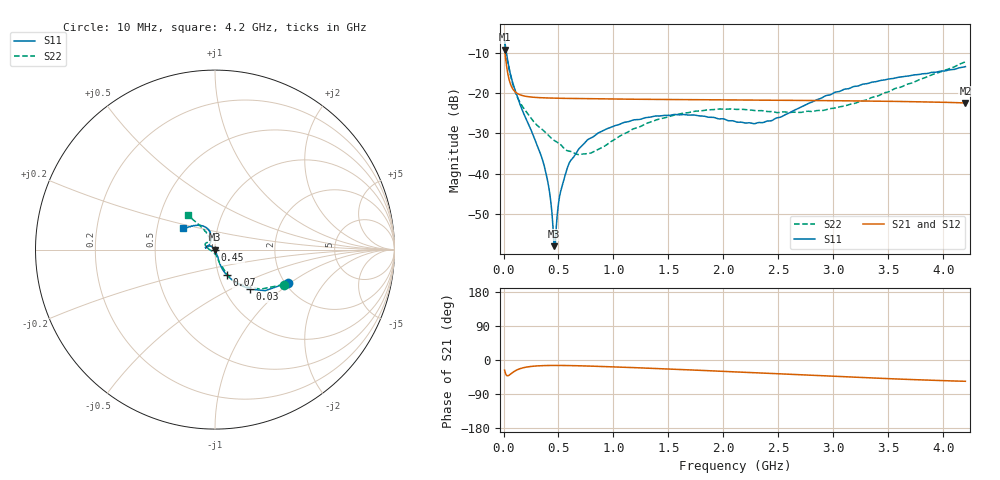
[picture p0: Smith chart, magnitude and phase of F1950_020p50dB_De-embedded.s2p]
! Integrated Device Technology
! Corporate Headquarters
! 6024 Silver Creek Valley Road
! San Jose, CA 95138  USA
! Phone:  1-408-284-8200
! Toll Free:  1-800-223-1366
! Webpage:  http://www.idt.com/
! Timing and RF Division
! 515 Groton Road, Suite 102
! Westford, MA 01886-6024
! Device:  F1950
! Description: 7-bit 0.25 dB Digital Step Attenuator
! Frequency:  150.0 -  4000.00 MHz
! Package:  4x4 mm Thin QFN Plastic Package: 24 pin
! Ports:  2 RF, 12 DC
!  Pin  1  = D0
!  Pin  2  = VDD
!  Pin  3  = Vmode
!  Pin  4  = GND
!  Pin  5  = RF1  =  Port 1
!  Pin  6  = GND
!  Pin  7  = GND
!  Pin  8  = GND
!  Pin  9  = GND
!  Pin 10  = GND
!  Pin 11  = GND
!  Pin 12  = GND
!  Pin 13  = GND
!  Pin 14  = RF2  =  Port 2
!  Pin 15  = GND
!  Pin 16  = LE
!  Pin 17  = CLK
!  Pin 18  = DATE
!  Pin 19  = D6
!  Pin 20  = D5
!  Pin 21  = D4
!  Pin 22  = D3
!  Pin 23  = D2
!  Pin 24  = D1
! State:  82
! Atten State:  20.50 dB
! Voltage:  +5.00 Volts
! Current:  Not Measured mA
! Data:  The device was measured on a the F195X evaluation board which has
!  individual transmission lines to the RF pins.  Data was collected
!  using a calibrated network analyzer.  The evaluation board was
!  de-embedded using a TRL calibration technique.
!  The reference plane is the edge of the package pin.
! Misc:  Board 2019
!  Action Tracker AT0250
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# GHz S dB R 50
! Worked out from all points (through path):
!   420 points, 10 MHz to 4.2 GHz, reference 50 ohm
!   highest |S21| = -9.25 dB at 10 MHz (marker M1); lowest = -22.5 dB at 4.2 GHz (marker M2)
!   group delay of S21, straight-line fit = 28.6 ps
!   lowest |S11| = -58.0 dB at 460 MHz (marker M3), VSWR 1.00, Z = 49.9 - j0.104 ohm
!   |S11| at or under -10 dB: 26.49 MHz to end of sweep
!   |S22| runs from -35.3 to -7.3 dB; largest |S21 - S12| = 0.00013
!   S11 on the Smith chart (normalised r, x): 10 MHz: 2.08, -0.96; 30 MHz: 1.31, -0.63; 70 MHz: 1.09, -0.32; 450 MHz: 1.00, -0.00; 4.2 GHz: 0.68, +0.17
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0.01  -6.98 -24.2  -9.25 -26.7  -9.24 -26.7  -7.35 -27.0
0.03  -10.63 -48.5  -13.71 -41.2  -13.71 -41.2  -11.22 -49.3
0.07  -16.09 -65.0  -18.25 -35.9  -18.25 -35.9  -16.39 -63.9
0.16  -23.51 -71.4  -20.53 -22.0  -20.53 -22.0  -22.80 -71.2
0.36  -37.08 -67.2  -21.19 -14.8  -21.19 -14.8  -29.22 -78.6
0.41  -43.11 -72.4  -21.24 -14.5  -21.24 -14.5  -30.52 -79.9
0.45  -53.25 -93.1  -21.27 -14.4  -21.27 -14.4  -31.54 -84.6
0.46  -57.96 -124.6  -21.28 -14.3  -21.28 -14.3  -31.74 -86.1
0.48  -53.15 151.7  -21.29 -14.3  -21.29 -14.3  -32.06 -88.7
0.5  -47.38 140.4  -21.30 -14.4  -21.30 -14.4  -32.38 -90.3
0.52  -44.34 138.5  -21.31 -14.4  -21.31 -14.4  -32.81 -91.5
0.57  -39.52 134.0  -21.33 -14.6  -21.33 -14.6  -34.16 -99.4
0.61  -36.76 135.9  -21.35 -14.8  -21.35 -14.8  -34.48 -107.3
0.71  -33.16 137.7  -21.39 -15.4  -21.39 -15.5  -35.16 -126.4
0.99  -28.34 147.6  -21.49 -18.1  -21.48 -18.1  -31.86 -172.4
1.41  -25.69 163.6  -21.59 -22.7  -21.59 -22.7  -26.50 165.1
1.73  -25.45 169.2  -21.66 -26.5  -21.65 -26.5  -24.56 156.4
2.11  -27.11 159.1  -21.73 -31.5  -21.73 -31.5  -24.05 146.9
2.43  -26.91 127.3  -21.79 -35.4  -21.79 -35.4  -24.60 136.9
2.81  -22.19 105.8  -21.87 -40.4  -21.86 -40.5  -24.56 121.8
3.51  -16.49 117.8  -22.05 -49.3  -22.05 -49.3  -19.62 116.8
4.2  -13.47 146.1  -22.46 -56.1  -22.46 -56.2  -12.27 128.4
